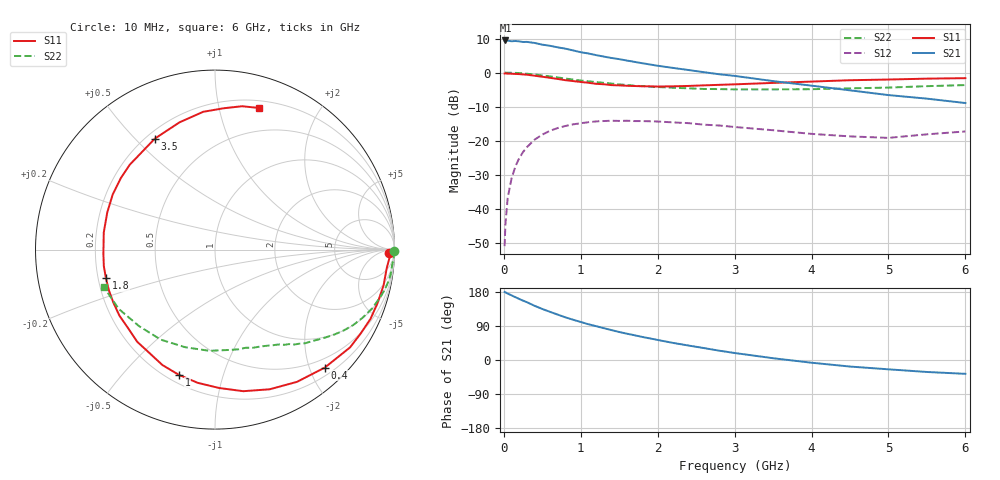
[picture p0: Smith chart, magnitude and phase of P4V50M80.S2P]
! SIEMENS Small Signal Semiconductors
! BFP182
! Si NPN RF Bipolar Junction Transistor in SOT143
! VCE = 0.5 V  IC = 0.8 mA
! Common Emitter S-Parameters:  March  1996
# GHz  S  MA  R  50
!  f  S11  S21  S12  S22
! GHz  MAG  ANG  MAG  ANG  MAG  ANG  MAG  ANG
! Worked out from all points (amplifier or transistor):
!   36 points, 10 MHz to 6 GHz, reference 50 ohm
!   highest |S21| = 9.4 dB at 20 MHz (marker M1)
!   |S21| within 3 dB of that: start of sweep to 914 MHz
!   unconditionally stable (mu >= 1): 2.522 GHz to end of sweep
!   at 250 MHz: K = 0.11, MSG = 16.2 dB, |S12| = -23.4 dB
!   at 1.4 GHz: K = 0.57, MSG = 9.2 dB, |S12| = -14.2 dB
!   at 6 GHz: K = 1.55, MAG = -0.2 dB, |S12| = -17.3 dB
!   S11 on the Smith chart (normalised r, x): 10 MHz: 43, -27; 400 MHz: 0.33, -2.25; 1 GHz: 0.24, -0.72; 1.8 GHz: 0.23, -0.12; 3.5 GHz: 0.23, +0.57; 6 GHz: 0.27, +1.32
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0.01  0.9676 -1.2  2.889 179.5  0.0028 88.6  0.9972 -0.5
0.02  0.9736 -2.6  2.961 178.8  0.0057 89.9  0.9958 -1.1
0.05  0.9625 -6.1  2.941 175.3  0.0143 87.0  0.9961 -2.7
0.1  0.9601 -11.9  2.883 170.6  0.0277 82.3  0.9903 -5.3
0.15  0.9535 -18.3  2.906 165.8  0.0416 78.3  0.9884 -8.1
0.3  0.9291 -35.9  2.819 152.5  0.08 66.9  0.9601 -15.7
0.4  0.8979 -47.1  2.722 143.0  0.103 59.6  0.9357 -20.4
0.6  0.8358 -68.6  2.472 127.1  0.1392 46.6  0.8777 -28.6
0.7  0.8045 -78.7  2.345 119.8  0.1527 41.0  0.8465 -32.2
0.8  0.7714 -88.3  2.244 112.6  0.1637 35.6  0.8165 -35.4
1  0.7265 -106.0  1.99 100.3  0.1798 26.2  0.7642 -40.9
1.1  0.7067 -114.5  1.904 94.3  0.1861 22.1  0.7427 -43.4
1.3  0.6719 -130.2  1.715 84.0  0.1936 14.3  0.7048 -48.0
1.5  0.6472 -145.4  1.573 73.9  0.1943 8.1  0.6687 -51.9
1.8  0.6283 -165.3  1.369 60.8  0.1933 0.6  0.6306 -57.2
2.2  0.6271 171.2  1.169 45.1  0.1848 -8.3  0.5962 -64.9
2.8  0.659 142.7  0.943 24.6  0.1664 -17.3  0.5707 -76.8
3.5  0.7035 118.4  0.748 4.7  0.1417 -21.8  0.5648 -93.3
4.5  0.7706 94.9  0.547 -17.3  0.1151 -17.3  0.5855 -121.0
5  0.7889 86.5  0.466 -24.6  0.1095 -8.1  0.6006 -134.7
5.5  0.8129 79.3  0.413 -31.6  0.1234 -2.8  0.6301 -148.4
6  0.8265 72.7  0.356 -36.5  0.1362 -1.2  0.6537 -161.3
